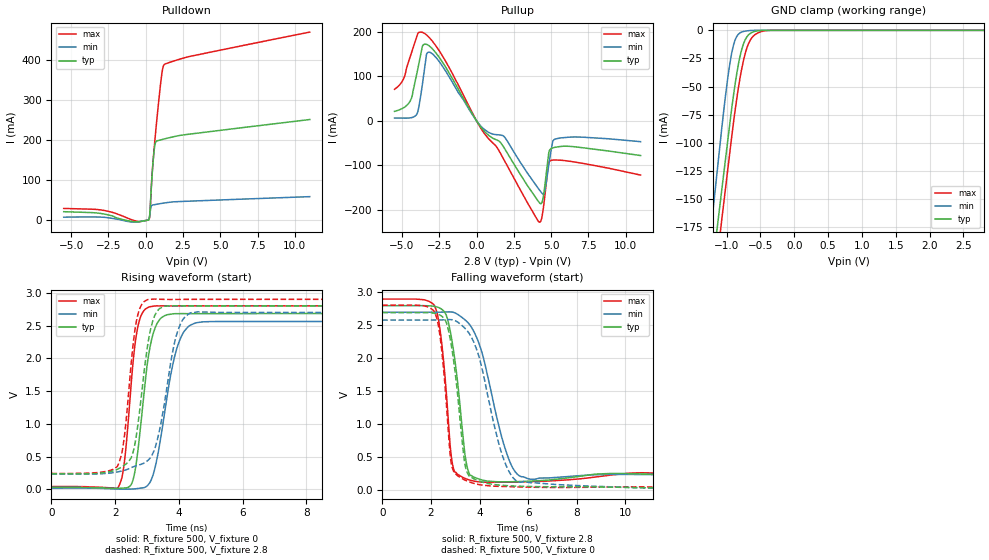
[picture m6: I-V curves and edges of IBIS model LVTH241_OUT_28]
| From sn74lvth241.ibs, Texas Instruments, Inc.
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[Model]   LVTH241_OUT_28
Model_type  3-state
Enable   Active-Low
Vref =   0
Rref =   500
Cref =   50p
Vmeas =   1.5
| variable   typ   min   max
C_comp   5.78pF   4.77pF   7.95pF
| C_pullup   4.83pF   0.31pF   7.53pF
| C_pulldown   6.03pF   1.99pF   10.06pF
| C_tri-state   5.78pF   4.77pF   7.95pF
[Temperature Range]   40   -40   100
| Ambient temperature   25   -40   85
[Voltage range]   2.8   2.7   2.9
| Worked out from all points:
|   slope of the pulldown table from 0 to 0.42 V, typ, clamps not added: 3.84 ohm
|   slope of the pullup table from 0 to 0.42 V, typ, clamps not added: 21.7 ohm
|   GND clamp passes 1 mA (typ) near -0.58 V on its own axis
|   rising waveform, R_fixture 500, V_fixture 0: 20-80 % time 382ps typ, 543ps min, 304ps max; typ from 0.032 V to 2.68 V
|   falling waveform, R_fixture 500, V_fixture 2.8: 20-80 % time 483ps typ, 981ps min, 372ps max; typ from 2.8 V to 0.238 V
|   rising waveform, R_fixture 500, V_fixture 2.8: 20-80 % time 408ps typ, 543ps min, 323ps max; typ from 0.238 V to 2.8 V
|   falling waveform, R_fixture 500, V_fixture 0: 20-80 % time 484ps typ, 995ps min, 376ps max; typ from 2.69 V to 0.032 V
[GND Clamp]
| LVTH241_OUT_28
|   Voltage   I(typ)   I(min)   I(max)
-5.5V     -2.834A    -3.019A    -2.865A
-1.25V    -230.6mA   -188.2mA   -259.6mA
-1.22V    -215.7mA   -171mA     -244mA
-1.18V    -195.7mA   -148.2mA   -223.3mA
-1.075V   -143.6mA   -88.9mA    -170mA
-975mV    -94.01mA   -38.87mA   -119.7mA
-925mV    -69.63mA   -20.27mA   -94.72mA
-875mV    -47.88mA   -8.568mA   -71.36mA
-800mV    -22.55mA   -2.203mA   -41.61mA
-725mV    -8.33mA    -701.6uA   -20.52mA
-575mV    -842.6uA   -11.41uA   -3.577mA
2.8V      28.19pA    20.95pA    1.196nA
[Pulldown]
| LVTH241_OUT_28
|   Voltage   I(typ)   I(min)   I(max)
-5.5V     21.78mA    8.121mA    29.98mA
-3.025V   17.44mA    8.251mA    26.21mA
-560mV    -3.717mA   -3.992mA   -2.565mA
195mV     1.392mA    1.507mA    1.436mA
285mV     22.67mA    17.64mA    18.47mA
365mV     76.4mA     34.67mA    76.09mA
465mV     132.9mA    38.47mA    134.9mA
620mV     189.6mA    39.58mA    203.1mA
1.03V     201.6mA    42.25mA    352.1mA
1.135V    202.7mA    42.89mA    379.1mA
1.23V     203.6mA    43.45mA    389.4mA
11V       252.3mA    59.42mA    471mA
[Pullup]
| LVTH241_OUT_28
|   Voltage   I(typ)   I(min)   I(max)
-5.5V     21.44mA    6.413mA    70.85mA
-4.465V   43.68mA    6.74mA     142.4mA
-3.99V    108.8mA    16.01mA    191mA
-3.62V    168.2mA    84.82mA    198.4mA
-3.245V   169.8mA    153.9mA    189.4mA
1.895V    -62.93mA   -36.94mA   -90.63mA
4.215V    -183.5mA   -154.8mA   -227.1mA
4.55V     -152.6mA   -160.2mA   -176.4mA
4.815V    -78.5mA    -105.1mA   -97.38mA
4.96V     -63.26mA   -73.72mA   -89.02mA
5.58V     -57.48mA   -38.47mA   -87.96mA
11V       -77.73mA   -46.53mA   -121.5mA
[Ramp]
| LVTH241_OUT_28
| variable   typ   min   max
dV/dt_r   1.60/3.90E-10   1.54/5.55E-10   1.67/3.11E-10
dV/dt_f   1.60/4.99E-10   1.51/1.02E-09   1.67/3.87E-10
R_load = 500
[Rising Waveform]
| LVTH241_OUT_28
R_fixture =   500
C_fixture =   0
L_fixture =   0
V_fixture =   0
V_fixture_min = 0
V_fixture_max = 0
|   Time   V(typ)   V(min)   V(max)
0s        32.2mV     19.9mV     45.21mV
2.075ns   16.01mV    5.976mV    21.24mV
2.285ns   21.83mV    3.951mV    401.6mV
2.5ns     70.65mV    5.395mV    1.598V
2.76ns    793.6mV    17.61mV    2.577V
3.015ns   1.939V     59.63mV    2.771V
3.24ns    2.445V     310.9mV    2.797V
3.96ns    2.68V      2.191V     2.799V
4.745ns   2.681V     2.556V     2.8V
50ns      2.684V     2.563V     2.801V
[Falling Waveform]
| LVTH241_OUT_28
R_fixture =   500
C_fixture =   0
L_fixture =   0
V_fixture =   2.8
V_fixture_min = 2.7
V_fixture_max = 2.9
|   Time   V(typ)   V(min)   V(max)
0s        2.8V       2.7V       2.9V
2.12ns    2.792V     2.701V     2.817V
2.35ns    2.766V     2.702V     2.505V
2.585ns   2.692V     2.704V     1.709V
2.94ns    2.096V     2.697V     318.9mV
3.455ns   421.7mV    2.568V     175.6mV
3.875ns   186.9mV    2.323V     135.6mV
5.2ns     132.1mV    479.4mV    126.7mV
6.11ns    141.7mV    169mV      133.7mV
50ns      237.6mV    231.9mV    243.7mV
[Rising Waveform]
| LVTH241_OUT_28
R_fixture =   500
C_fixture =   0
L_fixture =   0
V_fixture =   2.8
V_fixture_min = 2.7
V_fixture_max = 2.9
|   Time   V(typ)   V(min)   V(max)
0s        238mV      232.1mV    244.1mV
2.07ns    307.5mV    266.6mV    353.1mV
2.285ns   369mV      290.6mV    793.6mV
2.58ns    603.8mV    347.6mV    2.283V
2.765ns   1.189V     375.8mV    2.752V
3.055ns   2.307V     456.8mV    2.898V
3.365ns   2.746V     845.5mV    2.901V
3.96ns    2.801V     2.412V     2.898V
4.59ns    2.798V     2.709V     2.899V
50ns      2.8V       2.7V       2.9V
[Falling Waveform]
| LVTH241_OUT_28
R_fixture =   500
C_fixture =   0
L_fixture =   0
V_fixture =   0
V_fixture_min = 0
V_fixture_max = 0
|   Time   V(typ)   V(min)   V(max)
0s        2.695V     2.582V     2.808V
2.12ns    2.687V     2.583V     2.724V
2.345ns   2.662V     2.584V     2.415V
2.575ns   2.591V     2.586V     1.614V
2.885ns   2.094V     2.587V     335.3mV
3.43ns    345.6mV    2.445V     152.6mV
4.06ns    134.6mV    1.915V     84.4mV
4.925ns   78.86mV    546.5mV    60.87mV
5.66ns    64.19mV    124.8mV    53.24mV
50ns      32.23mV    19.91mV    45.26mV
